FUNCTION "APPOGGIO FC NC" : VOID
TITLE =
VERSION : 0.1

BEGIN
NETWORK
TITLE =Appoggio finecorsa con contatto normalmente chiuso
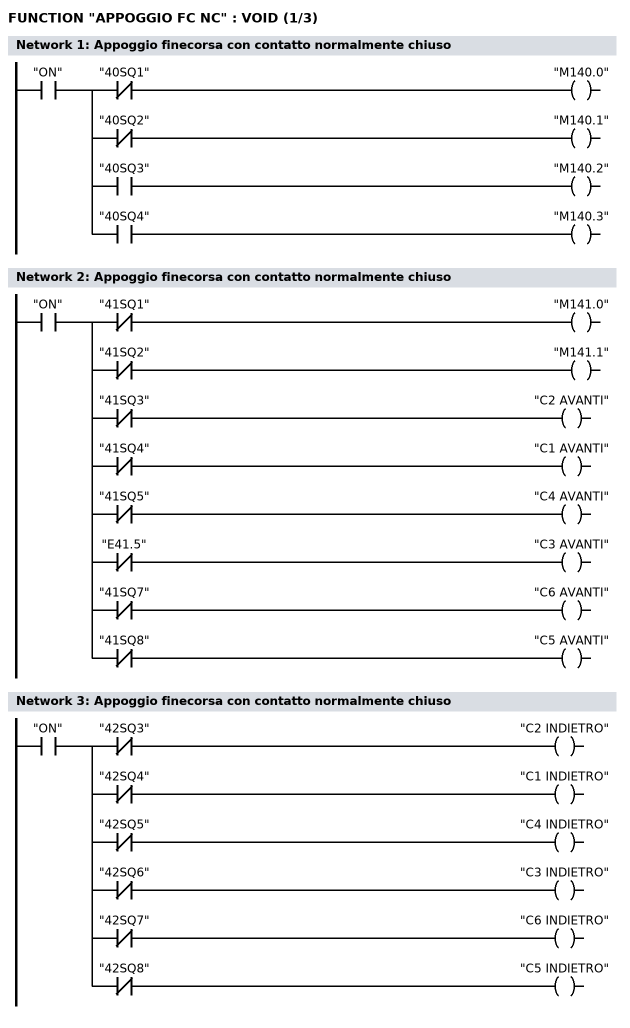
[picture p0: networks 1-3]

      U     "ON";
      =     L      0.0;
      U     L      0.0;
      UN    "40SQ1";
      =     "M140.0";
      U     L      0.0;
      UN    "40SQ2";
      =     "M140.1";
      U     L      0.0;
      U     "40SQ3";
      =     "M140.2";
      U     L      0.0;
      U     "40SQ4";
      =     "M140.3";
NETWORK
TITLE =Appoggio finecorsa con contatto normalmente chiuso

      U     "ON";
      =     L      0.0;
      U     L      0.0;
      UN    "41SQ1";
      =     "M141.0";
      U     L      0.0;
      UN    "41SQ2";
      =     "M141.1";
      U     L      0.0;
      UN    "41SQ3";
      =     "C2 AVANTI";
      U     L      0.0;
      UN    "41SQ4";
      =     "C1 AVANTI";
      U     L      0.0;
      UN    "41SQ5";
      =     "C4 AVANTI";
      U     L      0.0;
      UN    "E41.5";
      =     "C3 AVANTI";
      U     L      0.0;
      UN    "41SQ7";
      =     "C6 AVANTI";
      U     L      0.0;
      UN    "41SQ8";
      =     "C5 AVANTI";
NETWORK
TITLE =Appoggio finecorsa con contatto normalmente chiuso

      U     "ON";
      =     L      0.0;
      U     L      0.0;
      UN    "42SQ3";
      =     "C2 INDIETRO";
      U     L      0.0;
      UN    "42SQ4";
      =     "C1 INDIETRO";
      U     L      0.0;
      UN    "42SQ5";
      =     "C4 INDIETRO";
      U     L      0.0;
      UN    "42SQ6";
      =     "C3 INDIETRO";
      U     L      0.0;
      UN    "42SQ7";
      =     "C6 INDIETRO";
      U     L      0.0;
      UN    "42SQ8";
      =     "C5 INDIETRO";
NETWORK
TITLE =Appoggio finecorsa con contatto normalmente chiuso
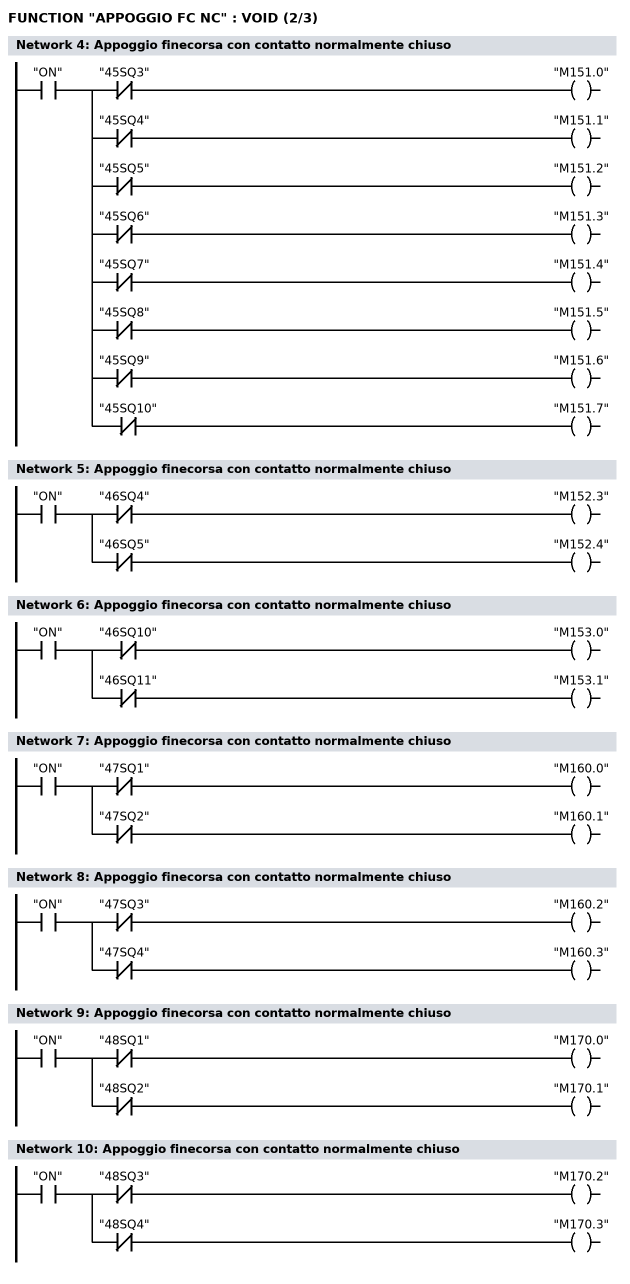
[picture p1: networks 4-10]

      U     "ON";
      =     L      0.0;
      U     L      0.0;
      UN    "45SQ3";
      =     "M151.0";
      U     L      0.0;
      UN    "45SQ4";
      =     "M151.1";
      U     L      0.0;
      UN    "45SQ5";
      =     "M151.2";
      U     L      0.0;
      UN    "45SQ6";
      =     "M151.3";
      U     L      0.0;
      UN    "45SQ7";
      =     "M151.4";
      U     L      0.0;
      UN    "45SQ8";
      =     "M151.5";
      U     L      0.0;
      UN    "45SQ9";
      =     "M151.6";
      U     L      0.0;
      UN    "45SQ10";
      =     "M151.7";
NETWORK
TITLE =Appoggio finecorsa con contatto normalmente chiuso

      U     "ON";
      =     L      0.0;
      U     L      0.0;
      UN    "46SQ4";
      =     "M152.3";
      U     L      0.0;
      UN    "46SQ5";
      =     "M152.4";
NETWORK
TITLE =Appoggio finecorsa con contatto normalmente chiuso

      U     "ON";
      =     L      0.0;
      U     L      0.0;
      UN    "46SQ10";
      =     "M153.0";
      U     L      0.0;
      UN    "46SQ11";
      =     "M153.1";
NETWORK
TITLE =Appoggio finecorsa con contatto normalmente chiuso

      U     "ON";
      =     L      0.0;
      U     L      0.0;
      UN    "47SQ1";
      =     "M160.0";
      U     L      0.0;
      UN    "47SQ2";
      =     "M160.1";
NETWORK
TITLE =Appoggio finecorsa con contatto normalmente chiuso

      U     "ON";
      =     L      0.0;
      U     L      0.0;
      UN    "47SQ3";
      =     "M160.2";
      U     L      0.0;
      UN    "47SQ4";
      =     "M160.3";
NETWORK
TITLE =Appoggio finecorsa con contatto normalmente chiuso

      U     "ON";
      =     L      0.0;
      U     L      0.0;
      UN    "48SQ1";
      =     "M170.0";
      U     L      0.0;
      UN    "48SQ2";
      =     "M170.1";
NETWORK
TITLE =Appoggio finecorsa con contatto normalmente chiuso

      U     "ON";
      =     L      0.0;
      U     L      0.0;
      UN    "48SQ3";
      =     "M170.2";
      U     L      0.0;
      UN    "48SQ4";
      =     "M170.3";
NETWORK
TITLE =Appoggio finecorsa con contatto normalmente chiuso
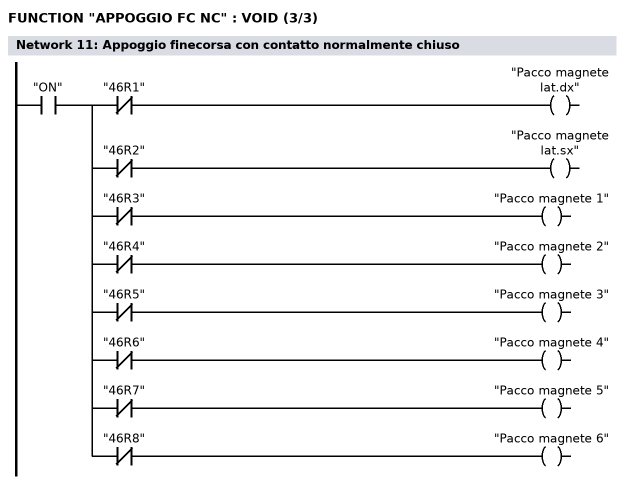
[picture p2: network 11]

      U     "ON";
      =     L      0.0;
      U     L      0.0;
      UN    "46R1";
      =     "Pacco magnete lat.dx";
      U     L      0.0;
      UN    "46R2";
      =     "Pacco magnete lat.sx";
      U     L      0.0;
      UN    "46R3";
      =     "Pacco magnete 1";
      U     L      0.0;
      UN    "46R4";
      =     "Pacco magnete 2";
      U     L      0.0;
      UN    "46R5";
      =     "Pacco magnete 3";
      U     L      0.0;
      UN    "46R6";
      =     "Pacco magnete 4";
      U     L      0.0;
      UN    "46R7";
      =     "Pacco magnete 5";
      U     L      0.0;
      UN    "46R8";
      =     "Pacco magnete 6";
END_FUNCTION

